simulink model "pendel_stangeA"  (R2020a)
settings: Solver=ode45  StartTime=0.0  StopTime=10  MaxStep=0.01  RelTol=1e-3  EnableMultiTasking=on
InitFcn:
  | init_pendelStange
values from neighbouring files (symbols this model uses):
  b = zeros(N, 1)    [fourierrechteck.m]    (also in init_lorenzC.m = 28; init_pendelStange.m = 0.2)
  g = 9.81    [init_pendelStange.m]
  l = 1    [init_pendelStange.m]    (also in sfun_pendelstangeanim.m = block.DialogPrm(2).Data)
  m = 1.0    (= 1)    [init_pendelStange.m]
  phi0 = 0.4*pi    (= 1.25663706144)    [init_pendelStange.m]

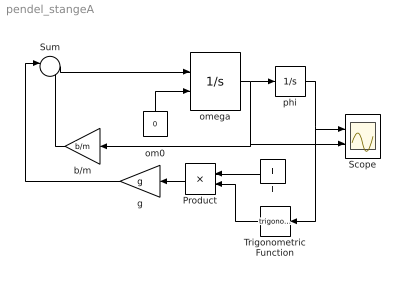
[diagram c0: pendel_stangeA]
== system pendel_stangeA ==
  note: .
  Product : Product  Inputs=/*  RndMeth=Zero
  Scope : Scope  NumInputPorts=2
  Sum : Sum  Inputs=|--  InputSameDT=on  SaturateOnIntegerOverflow=on
  Trigonometric Function : Trigonometry
  b/m : Gain  Gain=b/m  SaturateOnIntegerOverflow=on
  g : Gain  Gain=g  SaturateOnIntegerOverflow=on
  l : Constant  Value=l
  om0 : Constant  Value=0
  omega : Integrator  InitialConditionSource=external
  phi : Integrator  InitialCondition=phi0
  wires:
  omega/1 -> phi/1, b/m/1, Scope/2
  phi/1 -> Scope/1, Trigonometric Function/1
  Sum/1 -> omega/1
  b/m/1 -> Sum/2
  g/1 -> Sum/1
  Product/1 -> g/1
  om0/1 -> omega/2
  l/1 -> Product/1
  Trigonometric Function/1 -> Product/2
